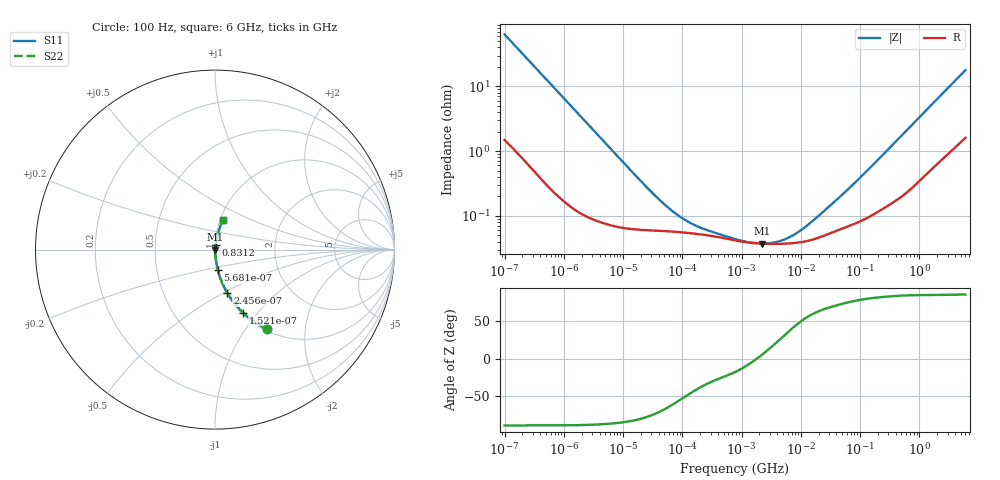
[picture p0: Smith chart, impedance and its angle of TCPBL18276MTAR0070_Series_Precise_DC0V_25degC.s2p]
! TCPBL18276MTAR0070 Polymer Tantalum Capacitor Sparameter Model
! Model Generated by Samsung Electro-Mechanics
! Samsung Sparameter Version 5.0
! Date : Oct-21-2025
! Products : Polymer Tantalum Capacitor
! Characteristics :
!  Nominal Capacitance = 27uF
!  Capacitance Tolerance = +/-20%
!  ESR = 70 mohm max at 100kHz
!  Rated Voltage = 18Vdc
!  Size = 1411(unit:inch), 3528(unit:mm)
!  Length = 3.50+/-0.20mm
!  Width = 2.80+/-0.20mm
!  Thickness = 1.10+/-0.10mm
!  Lineup = Conductive Polymer Type
!  Feature = PBL
!  Measurement Temperature : 25degC.
!  DC bias Value = 0V
!  Frequency : 100Hz ~ 6GHz
! External Node Assignments :
!  1  o---||---o  2
# MHz S RI R 50.0
! Freq.  Real(S11)  Im(S11)  Real(S12)  Im(S12)  Real(S21)  Im(S21)  Real(S22)  Im(S22)
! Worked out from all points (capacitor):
!   300 points, 100 Hz to 6 GHz, reference 50 ohm
!   read as one part in series: C = 25 uF near 106.2 Hz
!   lowest |Z| = 37.2 mohm at 2.21 MHz (marker M1)
!   series resonance near 1.82 MHz, so ESL is about 310 pH
!   S11 on the Smith chart (normalised r, x): 100 Hz: 1.03, -1.27; 152.1 Hz: 1.02, -0.84; 245.6 Hz: 1.01, -0.52; 568.1 Hz: 1.01, -0.23; 831.2 MHz: 1.01, +0.06; 6 GHz: 1.03, +0.36
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0.0001  0.2917 -0.443  0.7083 0.443  0.7083 0.443  0.2917 -0.443
0.0001520888  0.1561 -0.3512  0.8439 0.3512  0.8439 0.3512  0.1561 -0.3512
0.0002455886  0.0694 -0.2426  0.9306 0.2426  0.9306 0.2426  0.0694 -0.2426
0.000568071  0.0156 -0.1126  0.9844 0.1126  0.9844 0.1126  0.0156 -0.1126
0.001998454  0.00215 -0.0329  0.9979 0.0329  0.9979 0.0329  0.00215 -0.0329
0.01626223  0.000631 -0.00413  0.9994 0.00413  0.9994 0.00413  0.000631 -0.00413
0.03993819  0.000589 -0.00171  0.9994 0.00171  0.9994 0.00171  0.000589 -0.00171
0.07718646  0.000566 -0.000921  0.9994 0.000921  0.9994 0.000921  0.000566 -0.000921
0.1405012  0.000537 -0.000544  0.9995 0.000544  0.9995 0.000544  0.000537 -0.000544
0.2557518  0.000501 -0.000336  0.9995 0.000336  0.9995 0.000336  0.000501 -0.000336
0.7981464  0.000415 -0.00013  0.9996 0.00013  0.9996 0.00013  0.000415 -0.00013
1.368383  0.000384 -4.6e-05  0.9996 4.6e-05  0.9996 4.6e-05  0.000384 -4.6e-05
2.209625  0.000371 3.27e-05  0.9996 -3.27e-05  0.9996 -3.27e-05  0.000371 3.27e-05
3.56804  0.000367 0.000124  0.9996 -0.000124  0.9996 -0.000124  0.000367 0.000124
5.761569  0.000371 0.000245  0.9996 -0.000245  0.9996 -0.000245  0.000371 0.000245
9.303617  0.000387 0.000419  0.9996 -0.000419  0.9996 -0.000419  0.000387 0.000419
15.95059  0.000429 0.000719  0.9996 -0.000719  0.9996 -0.000719  0.000429 0.000719
63.25518  0.000694 0.00249  0.9993 -0.00249  0.9993 -0.00249  0.000694 0.00249
318.7652  0.00161 0.0112  0.9984 -0.0112  0.9984 -0.0112  0.00161 0.0112
831.1762  0.00368 0.0276  0.9963 -0.0276  0.9963 -0.0276  0.00368 0.0276
2593.922  0.0141 0.0791  0.9859 -0.0791  0.9859 -0.0791  0.0141 0.0791
6000  0.0449 0.167  0.9551 -0.167  0.9551 -0.167  0.0449 0.167
